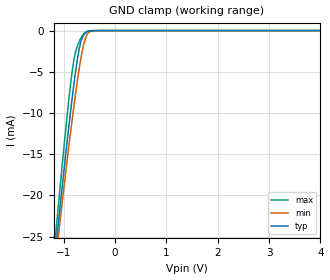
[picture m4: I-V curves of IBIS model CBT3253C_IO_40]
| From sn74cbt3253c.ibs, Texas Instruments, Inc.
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[Model]   CBT3253C_IO_40
Model_type  Terminator
| variable   typ   min   max
C_comp   13.43pF   11.24pF   17.82pF
| C_tri-state   13.43pF   11.24pF   17.82pF
[Temperature Range]   40   100   -40
| Ambient temperature   25   85   -40
[Voltage range]   4   4   4
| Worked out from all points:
|   GND clamp passes 1 mA (typ) near -0.65 V on its own axis
[GND Clamp]
| CBT3253C_IO_40
|   Voltage   I(typ)   I(min)   I(max)
-5V       -286.9mA   -267.5mA   -309.2mA
-1.175V   -27.56mA   -28.75mA   -25.86mA
-1.14V    -25.44mA   -26.81mA   -23.51mA
-1.105V   -23.33mA   -24.88mA   -21.17mA
-1.075V   -21.55mA   -23.24mA   -19.19mA
-920mV    -12.64mA   -15mA      -9.438mA
-815mV    -7.1mA     -9.759mA   -4.012mA
-685mV    -1.8mA     -4.053mA   -1.138mA
-610mV    -508.3uA   -1.615mA   -383.4uA
-550mV    -165.2uA   -531.9uA   -102.8uA
-325mV    -1.704uA   -7.127uA   -41.64nA
4V        782.8pA    2.221nA    355.9pA
